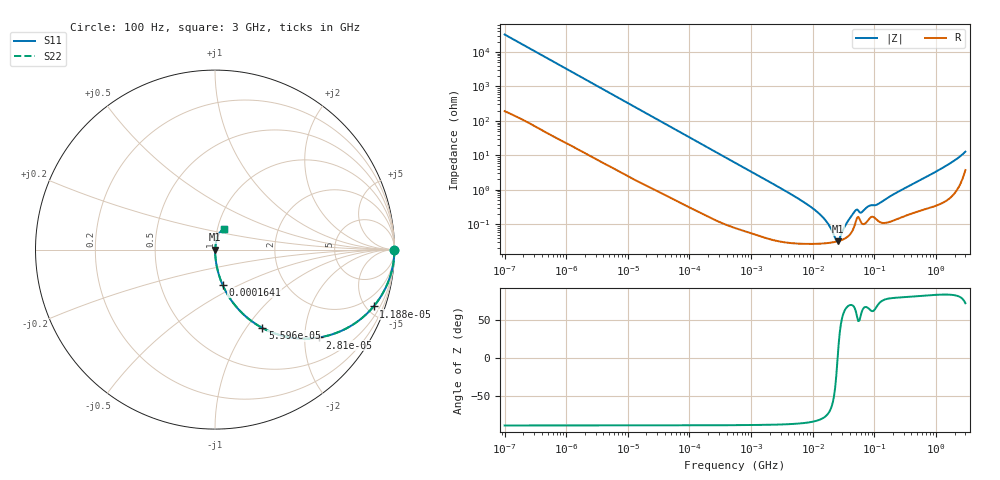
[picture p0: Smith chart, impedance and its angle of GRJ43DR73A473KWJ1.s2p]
!Murata Part Number: GRJ43DR73A473KWJ1
!These Parameters are Measured in Series Mode Connection
!Data Generated on Jun 19, 2026
!  o--ll--o
!Port1  Port2
!  o------o
!Operation Temp=25[degC], DC Bias Voltage=0[V]
!Freq. Start=100[Hz] Stop=3[GHz] 401[Steps]
# Hz S RI R 50
!Freq.(Hz) S11(Real) S11(Imag) S21(Real) S21(Imag) S12(Real) S12(Imag) S22(Real) S22(Imag)
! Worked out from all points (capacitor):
!   401 points, 100 Hz to 3 GHz, reference 50 ohm
!   read as one part in series: C = 49.2 nF near 109 Hz
!   lowest |Z| = 32 mohm at 25.25 MHz (marker M1)
!   series resonance near 25.32 MHz, so ESL is about 800 pH
!   S11 on the Smith chart (normalised r, x): 100 Hz: open; 11.88 kHz: 1.04, -5.56; 28.1 kHz: 1.02, -2.36; 55.95 kHz: 1.01, -1.19; 164.1 kHz: 1.00, -0.41; 3 GHz: 1.08, +0.25
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100  1 -0.00309  2.79e-05 0.00309  2.79e-05 0.00309  1 -0.00309
1788  0.9966 -0.0544  0.00335 0.0544  0.00335 0.0544  0.9966 -0.0544
5024  0.9762 -0.1488  0.0238 0.1488  0.0238 0.1488  0.9762 -0.1488
11882  0.8837 -0.3168  0.1163 0.3168  0.1163 0.3168  0.8837 -0.3168
28103  0.5818 -0.4891  0.4182 0.4891  0.4182 0.4891  0.5818 -0.4891
31977  0.5189 -0.4955  0.4811 0.4955  0.4811 0.4955  0.5189 -0.4955
55955  0.2636 -0.4362  0.7364 0.4362  0.7364 0.4362  0.2636 -0.4362
164120  0.0418 -0.1953  0.9582 0.1953  0.9582 0.1953  0.0418 -0.1953
547723  0.00454 -0.0612  0.9955 0.0612  0.9955 0.0612  0.00454 -0.0612
9794414  0.000278 -0.00297  0.9997 0.00297  0.9997 0.00297  0.000278 -0.00297
1.572531e7  0.000281 -0.00135  0.9997 0.00135  0.9997 0.00135  0.000281 -0.00135
2.316512e7  0.000308 -0.000246  0.9997 0.000246  0.9997 0.000246  0.000308 -0.000246
2.52476e7  0.00032 -8.3e-06  0.9997 8.3e-06  0.9997 8.3e-06  0.00032 -8.3e-06
2.751729e7  0.000334 0.000233  0.9997 -0.000233  0.9997 -0.000233  0.000334 0.000233
3.71925e7  0.000443 0.00115  0.9996 -0.00115  0.9996 -0.00115  0.000443 0.00115
4.815176e7  0.000965 0.00217  0.999 -0.00217  0.999 -0.00217  0.000965 0.00217
6.234031e7  0.00107 0.00196  0.9989 -0.00196  0.9989 -0.00196  0.00107 0.00196
8.070971e7  0.00138 0.00307  0.9986 -0.00307  0.9986 -0.00307  0.00138 0.00307
1.138854e8  0.00128 0.00361  0.9987 -0.00361  0.9987 -0.00361  0.00128 0.00361
1.751444e8  0.0012 0.00617  0.9988 -0.00617  0.9988 -0.00617  0.0012 0.00617
1.268426e9  0.00593 0.0424  0.9941 -0.0424  0.9941 -0.0424  0.00593 0.0424
3e9  0.0495 0.1125  0.9505 -0.1125  0.9505 -0.1125  0.0495 0.1125
